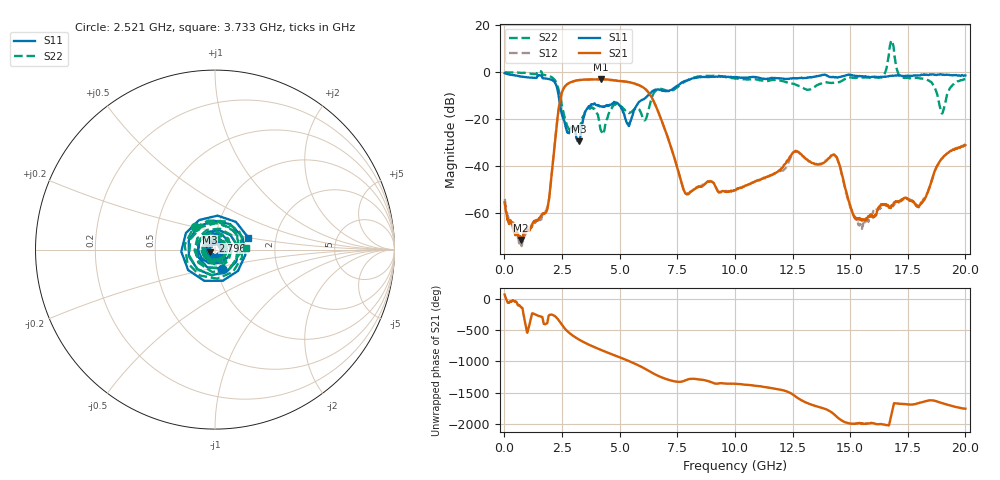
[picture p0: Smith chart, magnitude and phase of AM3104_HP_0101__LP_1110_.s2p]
!Created with skrf (http://scikit-rf.org).
# Hz S RI R 50.0
!freq ReS11 ImS11 ReS21 ImS21 ReS12 ImS12 ReS22 ImS22
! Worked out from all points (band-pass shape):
!   1601 points, 10 MHz to 20 GHz, reference 50 ohm
!   highest |S21| = -2.95 dB at 4.183 GHz (marker M1); lowest = -71.6 dB at 722.1 MHz (marker M2)
!   |S21| within 3 dB of the highest: 2.637 GHz to 5.932 GHz (3.295 GHz wide, 76.9 % of centre)
!   lowest |S11| = -29.4 dB at 3.221 GHz (marker M3), VSWR 1.07, Z = 47 - j1.39 ohm
!   |S11| at or under -10 dB: 2.352 GHz to 6.218 GHz (3.866 GHz wide, 90.2 % of centre)
!   |S22| runs from -26.5 to 13.6 dB; largest |S21 - S12| = 0.077
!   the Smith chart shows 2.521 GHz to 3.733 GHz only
!   S11 on the Smith chart (normalised r, x): 2.521 GHz: 1.06, -0.23; 2.796 GHz: 0.97, +0.10; 3.733 GHz: 1.44, +0.20
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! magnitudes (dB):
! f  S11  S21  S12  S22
! 10 MHz  -0.4  -55.4  -54.1  0.0
! 722.1 MHz  -1.8  -71.6  -73.5  -0.3
! 1.847 GHz  -2.8  -59.0  -58.1  -1.3
! 2.521 GHz  -18.9  -7.9  -8.0  -15.4
! 2.796 GHz  -25.8  -4.6  -4.7  -24.4
! 3.221 GHz  -29.4  -3.3  -3.4  -24.5
! 3.346 GHz  -23.9  -3.2  -3.3  -21.1
! 3.733 GHz  -14.1  -3.0  -3.1  -15.3
! 4.183 GHz  -14.6  -2.9  -3.0  -24.7
! 5.395 GHz  -23.0  -4.2  -4.2  -17.4
! 6.107 GHz  -11.0  -7.1  -7.2  -20.4
! 6.682 GHz  -7.3  -17.0  -17.1  -7.1
! 7.869 GHz  -3.7  -51.8  -51.4  -3.8
! 10.01 GHz  -2.2  -50.5  -50.6  -2.7
! 12.6 GHz  -2.6  -33.8  -33.8  -5.1
! 13.34 GHz  -2.2  -38.8  -38.6  -7.0
! 14.38 GHz  -2.1  -35.8  -36.0  -4.5
! 15.45 GHz  -1.7  -62.6  -64.9  -2.3
! 16.68 GHz  -1.7  -57.7  -57.2  7.3
! 18.03 GHz  -1.4  -56.8  -56.5  -2.7
! 18.98 GHz  -1.0  -36.9  -36.9  -17.5
! 20 GHz  -1.3  -31.2  -30.8  -2.9
